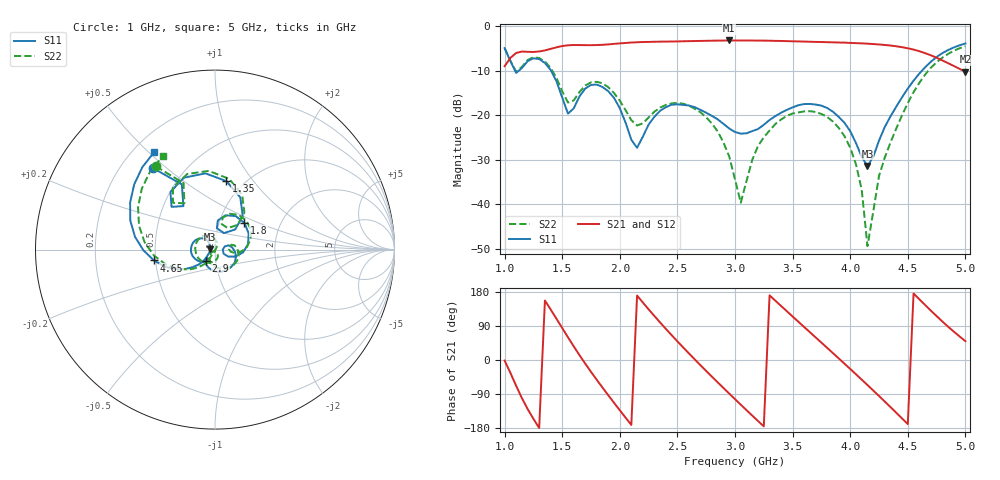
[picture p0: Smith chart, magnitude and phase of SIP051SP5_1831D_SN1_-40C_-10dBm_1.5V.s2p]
# GHz  S  dB  R  50
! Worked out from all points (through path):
!   81 points, 1 GHz to 5 GHz, reference 50 ohm
!   highest |S21| = -3.19 dB at 2.95 GHz (marker M1); lowest = -10.2 dB at 5 GHz (marker M2)
!   lowest |S11| = -31.4 dB at 4.15 GHz (marker M3), VSWR 1.06, Z = 47.4 + j0.242 ohm
!   |S11| at or under -10 dB: 1.091 GHz to 1.122 GHz (30.63 MHz wide, 2.77 % of centre); 1.404 GHz to 4.622 GHz (3.219 GHz wide, 107 % of centre)
!   |S22| runs from -49.4 to -4.5 dB; largest |S21 - S12| = 0.0022
!   S11 on the Smith chart (normalised r, x): 1 GHz: 0.34, +0.45; 1.35 GHz: 0.83, +0.75; 1.8 GHz: 1.32, +0.41; 2.9 GHz: 0.90, -0.11; 4.65 GHz: 0.49, -0.07; 5 GHz: 0.28, +0.52
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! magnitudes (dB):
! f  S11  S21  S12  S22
! 1 GHz  -4.9  -9.0  -9.0  -4.9
! 1.1 GHz  -10.5  -6.0  -6.0  -10.2
! 1.35 GHz  -8.2  -5.4  -5.4  -7.9
! 1.55 GHz  -19.6  -4.3  -4.3  -17.1
! 1.7 GHz  -14.0  -4.2  -4.2  -13.3
! 1.8 GHz  -13.1  -4.2  -4.2  -12.5
! 2.15 GHz  -27.3  -3.6  -3.6  -22.3
! 2.35 GHz  -19.0  -3.5  -3.5  -18.3
! 2.65 GHz  -18.2  -3.3  -3.3  -18.5
! 2.9 GHz  -21.9  -3.2  -3.2  -26.1
! 2.95 GHz  -23.0  -3.2  -3.2  -29.3
! 3 GHz  -23.8  -3.2  -3.2  -34.4
! 3.05 GHz  -24.1  -3.2  -3.2  -39.6
! 3.25 GHz  -22.1  -3.2  -3.2  -24.9
! 3.7 GHz  -17.6  -3.5  -3.5  -19.2
! 4 GHz  -23.6  -3.7  -3.7  -27.2
! 4.1 GHz  -29.3  -3.8  -3.8  -36.7
! 4.15 GHz  -31.4  -3.9  -3.9  -49.4
! 4.25 GHz  -25.7  -4.1  -4.1  -33.6
! 4.35 GHz  -20.2  -4.3  -4.3  -26.1
! 4.65 GHz  -9.2  -6.0  -6.0  -10.9
! 5 GHz  -3.9  -10.2  -10.2  -4.5
